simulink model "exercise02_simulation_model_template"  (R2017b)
settings: Solver=ode45  StartTime=0.0  StopTime=10  FixedStep=1e-5  MaxStep=1e-3  RelTol=1e-4  EnableMultiTasking=on
InitFcn:
  | exercise02_simulation_parameters
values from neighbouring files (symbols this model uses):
  cmd_2_newtons_conversion_linear_coefficient = 6.4870e-6    (= 6.487e-06)    [exercise02_get_crazyflie_inner_controller.m]
  cmd_2_newtons_conversion_quadratic_coefficient = 1.3385e-10    [exercise02_get_crazyflie_inner_controller.m]
  cmd_max = 2^16-1    (= 65535)    [exercise02_get_crazyflie_inner_controller.m]
  cmd_min = 0    [exercise02_get_crazyflie_inner_controller.m]
  g = 9.81    [exercise02_get_crazyflie_vehicle_paramters.m]
  K_lqr_outer_loop = K_lqr_outer_loop_discrete_time_200Hz    [exercise02_simulation_parameters.m]
  measurement_noise_accelerometer_covariance_decomposition = U * sqrt(D)    [exercise02_get_measurement_noise_details.m]
  measurement_noise_accelerometer_mean = zeros(3,1)    [exercise02_get_measurement_noise_details.m]
  measurement_noise_accelerometer_seed = randi(measurement_noise_randStream_for_seeds,2^32-1,3,1)    [exercise02_get_measurement_noise_details.m]
  measurement_noise_accelerometer_var = measurement_noise_accelerometer_stddev.^2    [exercise02_get_measurement_noise_details.m]
  measurement_noise_body_accelerations_inclusion_multiplier = 0    [exercise02_get_measurement_noise_details.m]
  measurement_noise_body_rates_inclusion_multiplier = 0    [exercise02_get_measurement_noise_details.m]
  measurement_noise_full_state_covariance_decomposition = U * sqrt(D)    [exercise02_get_measurement_noise_details.m]
  measurement_noise_full_state_inclusion_multiplier = 0    [exercise02_get_measurement_noise_details.m]
  measurement_noise_full_state_mean = [         measurement_noise_p_mean        ;         measurement_noise_p_dot_mean    ;         measurement_noise_psi_mean      ;         measurement_noise_psi_dot_mean        ]    [exercise02_get_measurement_noise_details.m]
  measurement_noise_full_state_seed = [         measurement_noise_p_seed        ;         measurement_noise_p_dot_seed    ;         measurement_noise_psi_seed      ;         measurement_noise_psi_dot_seed        ]    [exercise02_get_measurement_noise_details.m]
  measurement_noise_gyroscope_covariance_decomposition = U * sqrt(D)    [exercise02_get_measurement_noise_details.m]
  measurement_noise_gyroscope_mean = zeros(3,1)    [exercise02_get_measurement_noise_details.m]
  measurement_noise_gyroscope_seed = randi(measurement_noise_randStream_for_seeds,2^32-1,3,1)    [exercise02_get_measurement_noise_details.m]
  measurement_noise_gyroscope_var = measurement_noise_gyroscope_stddev.^2    [exercise02_get_measurement_noise_details.m]
  nrotor_initial_condition = [         nrotor_initial_condition_p          ;         nrotor_initial_condition_p_dot      ;         nrotor_initial_condition_psi        ;         nrotor_initial_condition_psi_dot    ;     ]    [exercise02_get_crazyflie_vehicle_paramters.m]
  nrotor_vehicle_equilibrium_thrust = exercise02_compute_equilibrium_thrusts(nrotor_vehicle_layout_for_controller,nrotor_vehicle_mass_for_controller,g)    [exercise02_simulation_parameters.m]
  nrotor_vehicle_inertia_true = [         16.57 ,   0.83 ,   0.72 ;          0.83 ,  16.66 ,   1.80 ;          0.72 ,   1.80 ,  29.26       ] * 1e-6    [exercise02_get_crazyflie_vehicle_paramters.m]
  nrotor_vehicle_inertia_true_inverse = inv(nrotor_vehicle_inertia_true)    [exercise02_get_crazyflie_vehicle_paramters.m]
  nrotor_vehicle_layout_true = [         [  1 , -1 , -1 ,  1 ] * x_baseline  ;         [ -1 , -1 ,  1 ,  1 ] * y_baseline  ;         [ -1 ,  1 , -1 ,  1 ] * c_baseline        ]    [exercise02_get_crazyflie_vehicle_paramters.m]
  nrotor_vehicle_mass_true = 32e-3    (= 0.032)    [exercise02_get_crazyflie_vehicle_paramters.m]
  nrotor_vehicle_thrust_max = 0.1597*ones( size(nrotor_vehicle_layout_true,2) , 1 )    [exercise02_get_crazyflie_vehicle_paramters.m]
  pid_x_body_rate_integrator_limit = 33.3    [exercise02_get_crazyflie_inner_controller.m]
  pid_x_body_rate_kp = 250.0    (= 250)    [exercise02_get_crazyflie_inner_controller.m]
  pid_y_body_rate_integrator_limit = 33.3    [exercise02_get_crazyflie_inner_controller.m]
  pid_y_body_rate_kp = 250.0    (= 250)    [exercise02_get_crazyflie_inner_controller.m]
  pid_z_body_rate_kp = 120.0    (= 120)    [exercise02_get_crazyflie_inner_controller.m]
  reference_saw_tooth_amplitude_xyz_yaw = [0.3; 0.3; 0.3; 3*deg2rad]    [exercise02_get_reference_specification.m]
  reference_saw_tooth_bias_xyz_yaw = [0.0; 0.0; 0.0; 0*deg2rad]    [exercise02_get_reference_specification.m]
  reference_saw_tooth_inclusion_multiplier = 0    [exercise02_get_reference_specification.m]
  reference_sine_amplitude_xyz_yaw = [0.3; 0.3; 0.3; 3*deg2rad]    [exercise02_get_reference_specification.m]
  reference_sine_bias_xyz_yaw = [0.0; 0.0; 0.0; 0*deg2rad]    [exercise02_get_reference_specification.m]
  reference_sine_period = 5    [exercise02_get_reference_specification.m]
  reference_sine_wave_inclusion_multiplier = 0    [exercise02_get_reference_specification.m]
  reference_step_inclusion_multiplier = 0    [exercise02_get_reference_specification.m]
  reference_step_period = 5    [exercise02_get_reference_specification.m]
  reference_step_xyz_yaw = [0.5; 0.5; 0.5; 10*deg2rad]    [exercise02_get_reference_specification.m]
  sample_time_controller_inner = 1/500    (= 0.002)    [exercise02_simulation_parameters.m]
  sample_time_controller_outer = 1/200    (= 0.005)    [exercise02_simulation_parameters.m]
  sample_time_measurements_body_accelerations = 1/500    (= 0.002)    [exercise02_simulation_parameters.m]
  sample_time_measurements_body_rates = 1/500    (= 0.002)    [exercise02_simulation_parameters.m]
  sample_time_measurements_full_state = 1/200    (= 0.005)    [exercise02_simulation_parameters.m]
undefined symbols (not defined in the file or in its folder): DiscIntNeverNeededParam, sigbuilder_block
libraries: simulink x3
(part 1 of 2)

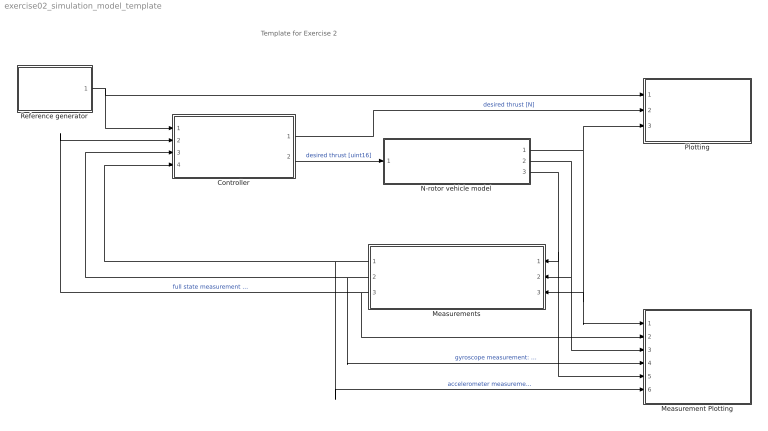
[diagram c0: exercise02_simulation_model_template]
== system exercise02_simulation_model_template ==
  note: Template for Exercise 2
  Controller : Subsystem
  Measurement Plotting : Subsystem
  Measurements : Subsystem
  N-rotor vehicle model : Subsystem
  Plotting : Subsystem
  Reference generator : Subsystem
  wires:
  Controller/1(thrust [N]) -> Plotting/2(thrusts)  "desired thrust [N]"
  N-rotor vehicle model/1(full state) -> Measurement Plotting/1(full state), Measurements/3(full state), Plotting/3(full state)
  Reference generator/1(x,y,z,yaw reference) -> Controller/1(reference), Plotting/1(reference)
  N-rotor vehicle model/2(body rates) -> Measurement Plotting/3(gyroscope), Measurements/2(body rates)
  N-rotor vehicle model/3(accelerations (body frame)) -> Measurement Plotting/5(accelerometer), Measurements/1(acceleration (body frame))
  Measurements/3(full state measurements) -> Controller/2(full state estimate), Measurement Plotting/2(full state measurements)  "full state measurement ( x,y,z , x_dot,y_dot,z_dot , roll,pitch,yaw , roll_dot,pitch_dot,yaw_dot )"
  Measurements/1(accelerometer measurements) -> Controller/4(body accelerations estimate), Measurement Plotting/6(accelerometer measurements)  "accelerometer measurement: ( x,y,z body accelerations )"
  Measurements/2(gyroscope measurements) -> Controller/3(body rates estimate), Measurement Plotting/4(gyroscope measurements)  "gyroscope measurement: ( x,y,z body rates )"
  Controller/2(cmd [uint16]) -> N-rotor vehicle model/1(cmd [uint16])  "desired thrust [uint16]"

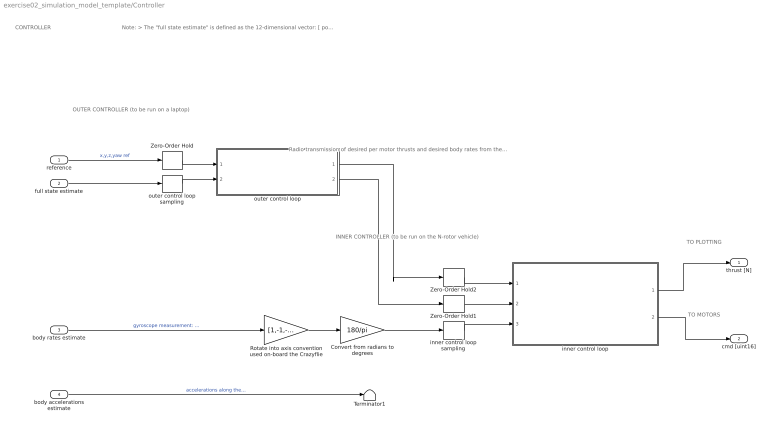
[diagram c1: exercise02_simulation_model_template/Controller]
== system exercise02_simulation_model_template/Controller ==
  note: CONTROLLER
  note: Note: > The "full state estimate" is defined as the 12-dimensional vector: [ position ; velocity ; euler angles ; euler rates ] > The "body rates estimate" is defined as a 3-dimensional vector: angular rate about the body frame [ x ; y ; z ] axes > The "body accelerations estimate" is defined as a 3-dimensional vector: acceleration along the body frame [ x ; y ; z ] axes > The "reference" input is as column vector of length four, specifying in order the reference for each of (x,y,z) position and the yaw euler angle. > The "per motor thrusts [N]" should be output as a column vector with length equal to the number of propellers on the vehicle, i.e., with length equal to N > The "per motor cmd [uint16]" should be output as a column vector with length equal to the number of propellers on the vehicle, i.e., with length equal to N
  note: TO PLOTTING
  note: TO MOTORS
  note: Radio transmission of desired per motor thrusts and desired body rates from the "off-board" laptop to the "on-baord" N-rotor vehicle's micro-processor
  note: OUTER CONTROLLER (to be run on a laptop)
  note: INNER CONTROLLER (to be run on the N-rotor vehicle)
  reference : Inport
  full state estimate : Inport  Port=2
  body rates estimate : Inport  Port=3
  body accelerations estimate : Inport  Port=4
  Convert from radians to degrees : Gain  Gain=180/pi
  Rotate into axis convention used on-board the Crazyflie : Gain  Gain=[1,-1,-1]
  Terminator1 : Terminator
  Zero-Order Hold : ZeroOrderHold  SampleTime=sample_time_controller_outer
  Zero-Order Hold1 : ZeroOrderHold  SampleTime=sample_time_controller_inner
  Zero-Order Hold2 : ZeroOrderHold  SampleTime=sample_time_controller_inner
  inner control loop sampling : ZeroOrderHold  SampleTime=sample_time_controller_inner
  inner control loop : Subsystem
  outer control loop sampling : ZeroOrderHold  SampleTime=sample_time_controller_outer
  outer control loop : Subsystem
  thrust [N] : Outport
  cmd [uint16] : Outport  Port=2
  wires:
  body accelerations estimate/1 -> Terminator1/1  "accelerations along the body frame (x,y,z) axes, in [m / second^2]"
  body rates estimate/1 -> Rotate into axis convention used on-board the Crazyflie/1  "gyroscope measurement: angular rates about the body frame (x,y,z) axes, in [radians / second]"
  inner control loop/1(per motor thrust [N]) -> thrust [N]/1
  reference/1 -> Zero-Order Hold/1  "x,y,z,yaw ref"
  inner control loop/2(per motor cmd [uint16]) -> cmd [uint16]/1
  outer control loop sampling/1 -> outer control loop/2(full state estimate)
  full state estimate/1 -> outer control loop sampling/1
  outer control loop/2(desired body rates [deg/s]) -> Zero-Order Hold1/1
  Rotate into axis convention used on-board the Crazyflie/1 -> Convert from radians to degrees/1
  outer control loop/1(desired per motor thrusts [uint16]) -> Zero-Order Hold2/1
  Convert from radians to degrees/1 -> inner control loop sampling/1
  Zero-Order Hold1/1 -> inner control loop/2(requested body rates [deg/s])
  Zero-Order Hold/1 -> outer control loop/1(reference)
  Zero-Order Hold2/1 -> inner control loop/1(requested per motor comand [uint16])
  inner control loop sampling/1 -> inner control loop/3(body rates estimate [deg/s])

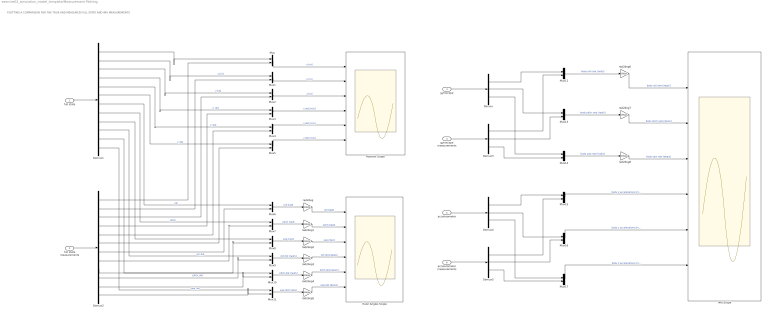
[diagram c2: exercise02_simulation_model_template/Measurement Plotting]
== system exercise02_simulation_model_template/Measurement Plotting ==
  note: PLOTTING A COMPARISON FOR THE TRUE AND MEASURED FULL STATE AND IMU MEASUREMENTS
  full state : Inport
  full state measurements : Inport  Port=2
  gyroscope : Inport  Port=3
  gyroscope measurements : Inport  Port=4
  accelerometer : Inport  Port=5
  accelerometer measurements : Inport  Port=6
  Demux{,3..5} (4 alike) : Demux  Outputs=3
  Demux1 : Demux  Outputs=12
  Demux2 : Demux  Outputs=12
  Euler Angles Scope : Scope  NumInputPorts=6
  IMU Scope : Scope  NumInputPorts=6
  Mux{,1..17} (18 alike) : Mux  Inputs=2
  Postiton Scope : Scope  NumInputPorts=6
  rad2deg{,1..8} (9 alike) : Gain  Gain=180/pi
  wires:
  full state/1 -> Demux1/1
  full state measurements/1 -> Demux2/1
  Mux/1 -> Postiton Scope/1  "x [m]"
  Mux1/1 -> Postiton Scope/2  "y [m]"
  Mux2/1 -> Postiton Scope/3  "z [m]"
  Mux3/1 -> Postiton Scope/4  "x dot [m/s]"
  Mux4/1 -> Postiton Scope/5  "y dot [m/s]"
  Mux5/1 -> Postiton Scope/6  "z dot [m/s]"
  Mux6/1 -> rad2deg/1  "roll [rad]"
  Mux7/1 -> rad2deg1/1  "pitch [rad]"
  Mux8/1 -> rad2deg2/1  "yaw [rad]"
  Mux9/1 -> rad2deg3/1  "roll dot [rad/s]"
  Mux10/1 -> rad2deg4/1  "pitch dot [rad/s]"
  Mux11/1 -> rad2deg5/1  "yaw dot [rad/s]"
  rad2deg/1 -> Euler Angles Scope/1  "roll [deg]"
  rad2deg2/1 -> Euler Angles Scope/3  "yaw [deg]"
  rad2deg1/1 -> Euler Angles Scope/2  "pitch [deg]"
  rad2deg3/1 -> Euler Angles Scope/4  "roll dot [deg/s]"
  rad2deg4/1 -> Euler Angles Scope/5  "pitch dot [deg/s]"
  rad2deg5/1 -> Euler Angles Scope/6  "yaw dot [deg/s]"
  Demux1/1 -> Mux/1
  Demux2/1 -> Mux/2
  Demux1/2 -> Mux1/1  "y [m]"
  Demux1/3 -> Mux2/1  "z [m]"
  Demux2/2 -> Mux1/2
  Demux2/3 -> Mux2/2
  Demux1/4 -> Mux3/1  "x_dot"
  Demux1/5 -> Mux4/1  "y_dot"
  Demux1/6 -> Mux5/1  "z_dot"
  Demux1/12 -> Mux11/1  "yaw_dot"
  Demux1/11 -> Mux10/1  "pitch_dot"
  Demux1/10 -> Mux9/1  "rol_dot"
  Demux1/9 -> Mux8/1
  Demux1/8 -> Mux7/1  "pitch"
  Demux1/7 -> Mux6/1  "roll"
  Demux2/4 -> Mux3/2
  Demux2/5 -> Mux4/2
  Demux2/6 -> Mux5/2
  Demux2/7 -> Mux6/2
  Demux2/8 -> Mux7/2
  Demux2/9 -> Mux8/2
  Demux2/10 -> Mux9/2
  Demux2/11 -> Mux10/2
  Demux2/12 -> Mux11/2
  gyroscope measurements/1 -> Demux3/1
  gyroscope/1 -> Demux/1
  Mux12/1 -> rad2deg6/1  "body roll rate [rad/s]"
  rad2deg6/1 -> IMU Scope/1  "body roll rate [deg/s]"
  Mux13/1 -> rad2deg7/1  "body pitch rate [rad/s]"
  rad2deg7/1 -> IMU Scope/2  "body pitch rate [deg/s]"
  Mux14/1 -> rad2deg8/1  "body yaw rate [rad/s]"
  rad2deg8/1 -> IMU Scope/3  "body yaw rate [deg/s]"
  Demux/1 -> Mux12/1
  Demux/2 -> Mux13/1
  Demux/3 -> Mux14/1
  Demux3/3 -> Mux14/2
  Demux3/2 -> Mux13/2
  Demux3/1 -> Mux12/2
  accelerometer measurements/1 -> Demux5/1
  accelerometer/1 -> Demux4/1
  Mux15/1 -> IMU Scope/4  "body x accelerations [m/s^2]"
  Mux16/1 -> IMU Scope/5  "body y accelerations [m/s^2]"
  Mux17/1 -> IMU Scope/6  "body z accelerations [m/s^2]"
  Demux4/1 -> Mux15/1
  Demux4/2 -> Mux16/1
  Demux4/3 -> Mux17/1
  Demux5/3 -> Mux17/2
  Demux5/2 -> Mux16/2
  Demux5/1 -> Mux15/2

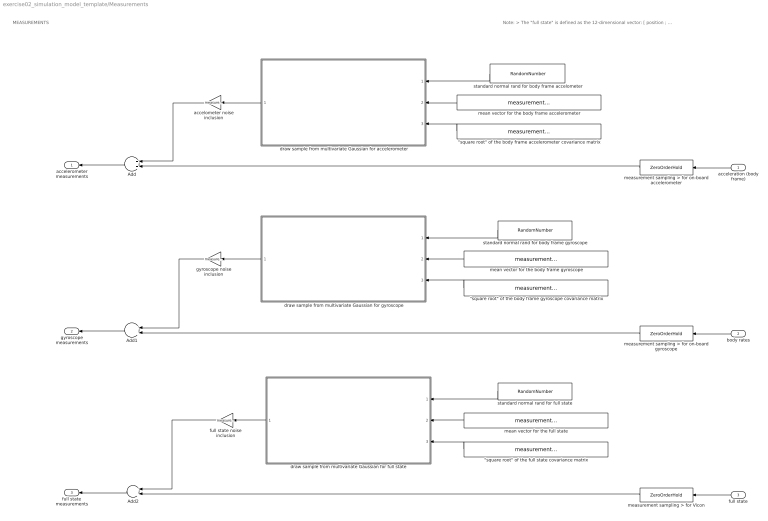
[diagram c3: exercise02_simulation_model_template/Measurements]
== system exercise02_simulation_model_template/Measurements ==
  note: Note: > The "full state" is defined as the 12-dimensional vector: [ position ; velocity ; euler angles ; euler rates ]
  note: MEASUREMENTS
  acceleration (body frame) : Inport
  body rates : Inport  Port=2
  full state : Inport  Port=3
  "\"square root\" of the body frame accelerometer covariance matrix" : Constant  Value=measurement_noise_accelerometer_covariance_decomposition
  "\"square root\" of the body frame gyroscope covariance matrix" : Constant  Value=measurement_noise_gyroscope_covariance_decomposition
  "\"square root\" of the full state covariance matrix" : Constant  Value=measurement_noise_full_state_covariance_decomposition
  Add : Sum
  Add1 : Sum
  Add2 : Sum
  accelometer noise inclusion : Gain  Gain=measurement_noise_body_accelerations_inclusion_multiplier
  draw sample from multivariate Gaussian for accelerometer : MATLAB Function  TreatAsAtomicUnit=on
  draw sample from multivariate Gaussian for full state : MATLAB Function  TreatAsAtomicUnit=on
  draw sample from multivariate Gaussian for gyroscope : MATLAB Function  TreatAsAtomicUnit=on
  full state noise inclusion : Gain  Gain=measurement_noise_full_state_inclusion_multiplier
  gyroscope noise inclusion : Gain  Gain=measurement_noise_body_rates_inclusion_multiplier
  mean vector for the body frame accelerometer : Constant  Value=measurement_noise_accelerometer_mean
  mean vector for the body frame gyroscope : Constant  Value=measurement_noise_gyroscope_mean
  mean vector for the full state : Constant  Value=measurement_noise_full_state_mean
  measurement sampling > for Vicon : ZeroOrderHold  SampleTime=sample_time_measurements_full_state
  measurement sampling > for on-board accelerometer : ZeroOrderHold  SampleTime=sample_time_measurements_body_accelerations
  measurement sampling > for on-board gyroscope : ZeroOrderHold  SampleTime=sample_time_measurements_body_rates
  standard normal rand for body frame accelometer : RandomNumber  Mean=measurement_noise_accelerometer_mean  Variance=measurement_noise_accelerometer_var  Seed=measurement_noise_accelerometer_seed  SampleTime=sample_time_measurements_body_accelerations  VectorParams1D=off
  standard normal rand for body frame gyroscope : RandomNumber  Mean=measurement_noise_gyroscope_mean  Variance=measurement_noise_gyroscope_var  Seed=measurement_noise_gyroscope_seed  SampleTime=sample_time_measurements_body_rates  VectorParams1D=off
  standard normal rand for full state : RandomNumber  Mean=zeros(12,1)  Variance=ones(12,1)  Seed=measurement_noise_full_state_seed  SampleTime=sample_time_measurements_full_state  VectorParams1D=off
  accelerometer measurements : Outport
  gyroscope measurements : Outport  Port=2
  full state measurements : Outport  Port=3
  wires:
  full state/1 -> measurement sampling > for Vicon/1
  acceleration (body frame)/1 -> measurement sampling > for on-board accelerometer/1
  body rates/1 -> measurement sampling > for on-board gyroscope/1
  measurement sampling > for Vicon/1 -> Add2/2
  "\"square root\" of the full state covariance matrix"/1 -> draw sample from multivariate Gaussian for full state/3(covariance_matrix_decomposition)
  mean vector for the full state/1 -> draw sample from multivariate Gaussian for full state/2(mean_vector)
  mean vector for the body frame gyroscope/1 -> draw sample from multivariate Gaussian for gyroscope/2(mean_vector)
  gyroscope noise inclusion/1 -> Add1/1
  measurement sampling > for on-board accelerometer/1 -> Add/2
  mean vector for the body frame accelerometer/1 -> draw sample from multivariate Gaussian for accelerometer/2(mean_vector)
  draw sample from multivariate Gaussian for accelerometer/1(rand_sample) -> accelometer noise inclusion/1
  draw sample from multivariate Gaussian for gyroscope/1(rand_sample) -> gyroscope noise inclusion/1
  standard normal rand for full state/1 -> draw sample from multivariate Gaussian for full state/1(std_normal_rand_sample)
  "\"square root\" of the body frame gyroscope covariance matrix"/1 -> draw sample from multivariate Gaussian for gyroscope/3(covariance_matrix_decomposition)
  accelometer noise inclusion/1 -> Add/1
  draw sample from multivariate Gaussian for full state/1(rand_sample) -> full state noise inclusion/1
  full state noise inclusion/1 -> Add2/1
  measurement sampling > for on-board gyroscope/1 -> Add1/2
  standard normal rand for body frame gyroscope/1 -> draw sample from multivariate Gaussian for gyroscope/1(std_normal_rand_sample)
  standard normal rand for body frame accelometer/1 -> draw sample from multivariate Gaussian for accelerometer/1(std_normal_rand_sample)
  Add2/1 -> full state measurements/1
  "\"square root\" of the body frame accelerometer covariance matrix"/1 -> draw sample from multivariate Gaussian for accelerometer/3(covariance_matrix_decomposition)
  Add/1 -> accelerometer measurements/1
  Add1/1 -> gyroscope measurements/1

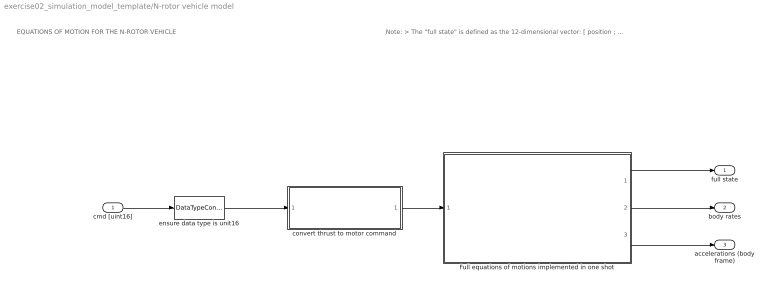
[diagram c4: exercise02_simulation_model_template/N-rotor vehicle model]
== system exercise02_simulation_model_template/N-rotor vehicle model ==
  note: Note: > The "full state" is defined as the 12-dimensional vector: [ position ; velocity ; euler angles ; euler rates ] > The "thrust [N]" input should be a column vector with length equal to the number of propellers on the vehicle, i.e., with length equal to N
  note: EQUATIONS OF MOTION FOR THE N-ROTOR VEHICLE
  cmd [uint16] : Inport
  Full equations of motions implemented in one shot : Subsystem
  convert thrust to motor command : Subsystem
  ensure data type is unit16 : DataTypeConversion  OutDataTypeStr=uint16
  full state : Outport
  body rates : Outport  Port=2
  accelerations (body frame) : Outport  Port=3
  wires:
  cmd [uint16]/1 -> ensure data type is unit16/1
  Full equations of motions implemented in one shot/1(full state) -> full state/1
  Full equations of motions implemented in one shot/2(body rates) -> body rates/1
  Full equations of motions implemented in one shot/3(body accellerations) -> accelerations (body frame)/1
  convert thrust to motor command/1(thrust [N]) -> Full equations of motions implemented in one shot/1(thrusts [N])
  ensure data type is unit16/1 -> convert thrust to motor command/1(cmd [uint16])

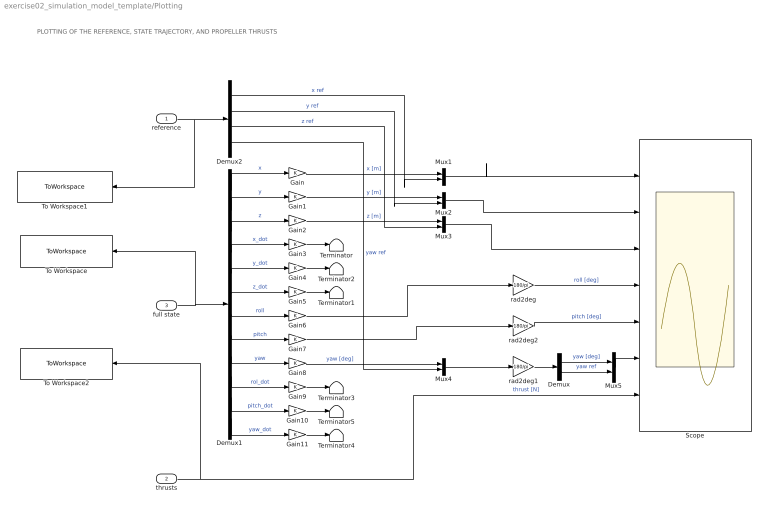
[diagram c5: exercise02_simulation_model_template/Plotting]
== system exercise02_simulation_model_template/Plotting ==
  note: PLOTTING OF THE REFERENCE, STATE TRAJECTORY, AND PROPELLER THRUSTS
  reference : Inport
  thrusts : Inport  Port=2
  full state : Inport  Port=3
  Demux : Demux  Outputs=2
  Demux1 : Demux  Outputs=12
  Demux2 : Demux
  Gain{,1..11} (12 alike) : Gain
  Mux{1..5} (5 alike) : Mux  Inputs=2
  Scope : Scope  NumInputPorts=7
  Terminator{,1..5} (6 alike) : Terminator
  To Workspace : ToWorkspace  VariableName=simout_full_state  SaveFormat=Timeseries  SampleTime=-1
  To Workspace1 : ToWorkspace  VariableName=simout_reference  SaveFormat=Timeseries  SampleTime=-1
  To Workspace2 : ToWorkspace  VariableName=simout_thrusts  SaveFormat=Timeseries  SampleTime=-1
  rad2deg : Gain  Gain=180/pi
  rad2deg1 : Gain  Gain=180/pi
  rad2deg2 : Gain  Gain=180/pi
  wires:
  Demux1/1 -> Gain/1  "x"
  Demux1/2 -> Gain1/1  "y"
  Demux1/6 -> Gain5/1  "z_dot"
  Gain7/1 -> rad2deg2/1
  Demux1/8 -> Gain7/1  "pitch"
  full state/1 -> To Workspace/1, Demux1/1
  Demux1/5 -> Gain4/1  "y_dot"
  Demux1/7 -> Gain6/1  "roll"
  Demux1/4 -> Gain3/1  "x_dot"
  Demux1/3 -> Gain2/1  "z"
  Gain6/1 -> rad2deg/1
  Demux1/9 -> Gain8/1  "yaw"
  Demux1/10 -> Gain9/1  "rol_dot"
  Demux1/11 -> Gain10/1  "pitch_dot"
  Demux1/12 -> Gain11/1  "yaw_dot"
  Gain9/1 -> Terminator3/1
  Gain10/1 -> Terminator5/1
  Gain11/1 -> Terminator4/1
  Gain3/1 -> Terminator/1
  Gain4/1 -> Terminator2/1
  Gain5/1 -> Terminator1/1
  thrusts/1 -> To Workspace2/1, Scope/7  "thrust [N]"
  reference/1 -> To Workspace1/1, Demux2/1
  Mux1/1 -> Scope/1
  Mux2/1 -> Scope/2
  Gain/1 -> Mux1/1  "x [m]"
  Demux2/1 -> Mux1/2  "x ref"
  Gain1/1 -> Mux2/1  "y [m]"
  Demux2/2 -> Mux2/2  "y ref"
  Mux3/1 -> Scope/3
  Gain2/1 -> Mux3/1  "z [m]"
  Demux2/3 -> Mux3/2  "z ref"
  Mux4/1 -> rad2deg1/1
  Gain8/1 -> Mux4/1  "yaw [deg]"
  Demux2/4 -> Mux4/2  "yaw ref"
  rad2deg/1 -> Scope/4  "roll [deg]"
  rad2deg2/1 -> Scope/5  "pitch [deg]"
  Demux/1 -> Mux5/1  "yaw [deg]"
  Demux/2 -> Mux5/2  "yaw ref"
  rad2deg1/1 -> Demux/1
  Mux5/1 -> Scope/6

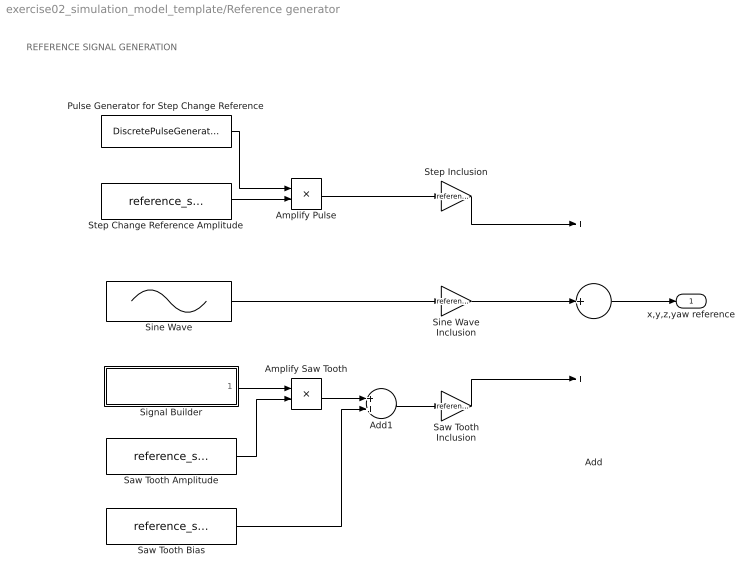
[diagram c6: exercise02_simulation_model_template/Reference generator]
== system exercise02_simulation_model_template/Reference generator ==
  note: REFERENCE SIGNAL GENERATION
  Add : Sum  Inputs=+++
  Add1 : Sum
  Amplify Pulse : Product
  Amplify Saw Tooth : Product
  Pulse Generator for Step Change Reference : DiscretePulseGenerator  PulseType=Time based  Period=reference_step_period*2  PulseWidth=50
  Saw Tooth Amplitude : Constant  Value=reference_saw_tooth_amplitude_xyz_yaw
  Saw Tooth Bias : Constant  Value=reference_saw_tooth_bias_xyz_yaw
  Saw Tooth Inclusion : Gain  Gain=reference_saw_tooth_inclusion_multiplier
  Signal Builder : Subsystem  Tag=STV Subsys  LoadFcn=sigbuilder_block('load');  StartFcn=sigbuilder_block('start');  StopFcn=sigbuilder_block('stop');  ClipboardFcn=sigbuilder_block('clipboard');  mask(Sigbuilder block){tuvar=[0:10]}
      mask help: Simulink:masks:SigbuilderBlock_MD
      mask init:
      | if ~strcmp(get_param(bdroot(gcbh),'SimulationStatus'),'stopped') tuvar = sigbuilder_block('maskInit'); end
  Sine Wave : Sin  Amplitude=reference_sine_amplitude_xyz_yaw  Bias=reference_sine_bias_xyz_yaw  Frequency=2*pi()/reference_sine_period  SampleTime=0
  Sine Wave Inclusion : Gain  Gain=reference_sine_wave_inclusion_multiplier
  Step Change Reference Amplitude : Constant  Value=reference_step_xyz_yaw
  Step Inclusion : Gain  Gain=reference_step_inclusion_multiplier
  x,y,z,yaw reference : Outport
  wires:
  Step Change Reference Amplitude/1 -> Amplify Pulse/2
  Pulse Generator for Step Change Reference/1 -> Amplify Pulse/1
  Sine Wave/1 -> Sine Wave Inclusion/1
  Add/1 -> x,y,z,yaw reference/1
  Step Inclusion/1 -> Add/1
  Sine Wave Inclusion/1 -> Add/2
  Amplify Pulse/1 -> Step Inclusion/1
  Saw Tooth Inclusion/1 -> Add/3
  Signal Builder/1(Saw Tooth) -> Amplify Saw Tooth/1
  Saw Tooth Amplitude/1 -> Amplify Saw Tooth/2
  Amplify Saw Tooth/1 -> Add1/1
  Add1/1 -> Saw Tooth Inclusion/1
  Saw Tooth Bias/1 -> Add1/2

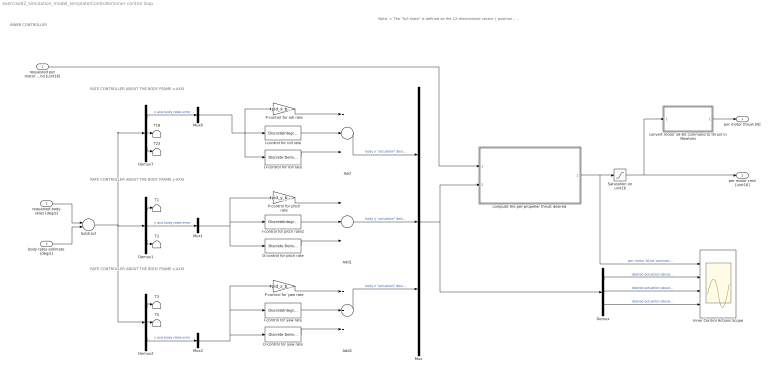
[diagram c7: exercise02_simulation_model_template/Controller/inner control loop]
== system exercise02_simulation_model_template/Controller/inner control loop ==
  note: RATE CONTROLLER ABOUT THE BODY FRAME z-AXIS
  note: RATE CONTROLLER ABOUT THE BODY FRAME y-AXIS
  note: RATE CONTROLLER ABOUT THE BODY FRAME x-AXIS
  note: INNER CONTROLLER
  note: Note: > The "full state" is defined as the 12-dimensional vector: [ position ; velocity ; euler angles ; euler rates ] > The "thrusts ref" is input as a column vector with a desired 16-bit command per motor, i.e., with length equal to N
  requested per motor comand [uint16] : Inport
  requested body rates [deg/s] : Inport  Port=2
  body rates estimate [deg/s] : Inport  Port=3
  Add : Sum  Inputs=+++
  Add1 : Sum  Inputs=+++
  Add2 : Sum  Inputs=+++
  D-control for pitch rate : simulink/Discrete/Discrete Derivative  gainval=pid_y_body_rate_kd  ICPrevScaledInput=0.0  OutMin=[]  OutMax=[]  OutDataType=fixdt(1, 16)  OutScaling=2^-10  DoSatur=off
  D-control for roll rate : simulink/Discrete/Discrete Derivative  gainval=pid_x_body_rate_kd  ICPrevScaledInput=0.0  OutMin=[]  OutMax=[]  OutDataType=fixdt(1, 16)  OutScaling=2^-10  DoSatur=off
  D-control for yaw rate : simulink/Discrete/Discrete Derivative  gainval=pid_z_body_rate_kd  ICPrevScaledInput=0.0  OutMin=[]  OutMax=[]  OutDataType=fixdt(1, 16)  OutScaling=2^-10  DoSatur=off
  Demux{,1..2,7} (4 alike) : Demux  Outputs=3
  I-control for pitch rate2 : DiscreteIntegrator  gainval=pid_y_body_rate_ki  InitialConditionSetting=State (most efficient)  SampleTime=-1  LimitOutput=on  UpperSaturationLimit=pid_y_body_rate_integrator_limit  LowerSaturationLimit=-pid_y_body_rate_integrator_limit  ICPrevOutput=DiscIntNeverNeededParam  ICPrevScaledInput=DiscIntNeverNeededParam
  I-control for roll rate : DiscreteIntegrator  gainval=pid_x_body_rate_ki  InitialConditionSetting=State (most efficient)  SampleTime=-1  LimitOutput=on  UpperSaturationLimit=pid_x_body_rate_integrator_limit  LowerSaturationLimit=-pid_x_body_rate_integrator_limit  ICPrevOutput=DiscIntNeverNeededParam  ICPrevScaledInput=DiscIntNeverNeededParam
  I-control for yaw rate : DiscreteIntegrator  gainval=pid_z_body_rate_ki  InitialConditionSetting=State (most efficient)  SampleTime=-1  LimitOutput=on  UpperSaturationLimit=pid_x_body_rate_integrator_limit  LowerSaturationLimit=-pid_x_body_rate_integrator_limit  ICPrevOutput=DiscIntNeverNeededParam  ICPrevScaledInput=DiscIntNeverNeededParam
  Inner Control Actions Scope : Scope  NumInputPorts=4
  Mux : Mux  Inputs=3
  Mux1 : Mux  Inputs=1
  Mux2 : Mux  Inputs=1
  Mux6 : Mux  Inputs=1
  P-control for pitch rate : Gain  Gain=pid_y_body_rate_kp
  P-control for roll rate : Gain  Gain=pid_x_body_rate_kp
  P-control for yaw rate : Gain  Gain=pid_z_body_rate_kp
  Saturation on uint16 : Saturate  UpperLimit=cmd_max  LowerLimit=cmd_min  ZeroCross=off
  Subtract : Sum  Inputs=+-
  T{1..3,5,18,23} (6 alike) : Terminator
  compute the per-propeller thrust desired : MATLAB Function  TreatAsAtomicUnit=on
  convert motor 16-bit command to thrust in Newtons : Subsystem
  per motor thrust [N] : Outport
  per motor cmd [uint16] : Outport  Port=2
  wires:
  compute the per-propeller thrust desired/1(cmd_to_apply) -> Inner Control Actions Scope/1, Saturation on uint16/1  "per motor 16-bit command after distribute power function [uint16]"
  body rates estimate [deg/s]/1 -> Subtract/2
  requested per motor comand [uint16]/1 -> compute the per-propeller thrust desired/1(cmd_per_motor_desired)
  requested body rates [deg/s]/1 -> Subtract/1
  Add/1 -> Mux/1  "body x \"actuation\" desired [uint16]"
  Add1/1 -> Mux/2  "body y \"actuation\" desired [uint16]"
  Add2/1 -> Mux/3  "body z \"actuation\" desired [uint16]"
  Subtract/1 -> Demux2/1, Demux1/1, Demux7/1
  Mux/1 -> Demux/1, compute the per-propeller thrust desired/2(cmd_for_body_torques_desired)
  Saturation on uint16/1 -> per motor cmd [uint16]/1, convert motor 16-bit command to thrust in Newtons/1(cmd [uint16])
  Demux/1 -> Inner Control Actions Scope/2  "desired actuation about body frame x axis [uint16]"
  Demux/2 -> Inner Control Actions Scope/3  "desired actuation about body frame x axis [uint16]"
  Demux/3 -> Inner Control Actions Scope/4  "desired actuation about body frame x axis [uint16]"
  Demux7/2 -> T18/1
  Mux6/1 -> P-control for roll rate/1, I-control for roll rate/1, D-control for roll rate/1
  Demux7/3 -> T23/1
  Demux7/1 -> Mux6/1  "x axis body rates error"
  Demux1/2 -> Mux1/1  "y axis body rates error"
  Demux1/3 -> T2/1
  Demux1/1 -> T1/1
  Demux2/3 -> Mux2/1  "z axis body rates error"
  Demux2/1 -> T3/1
  Mux2/1 -> I-control for yaw rate/1, P-control for yaw rate/1, D-control for yaw rate/1
  Demux2/2 -> T5/1
  convert motor 16-bit command to thrust in Newtons/1(thrusts [N]) -> per motor thrust [N]/1
  P-control for roll rate/1 -> Add/1
  I-control for roll rate/1 -> Add/2
  D-control for roll rate/1 -> Add/3
  P-control for pitch rate/1 -> Add1/1
  I-control for pitch rate2/1 -> Add1/2
  D-control for pitch rate/1 -> Add1/3
  Mux1/1 -> D-control for pitch rate/1, P-control for pitch rate/1, I-control for pitch rate2/1
  D-control for yaw rate/1 -> Add2/3
  P-control for yaw rate/1 -> Add2/1
  I-control for yaw rate/1 -> Add2/2

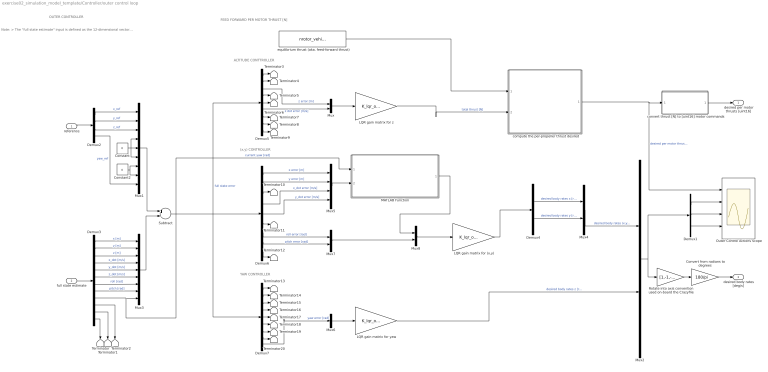
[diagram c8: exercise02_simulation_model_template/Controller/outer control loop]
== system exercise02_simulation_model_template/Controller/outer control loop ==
  note: FEED FORWARD PER MOTOR THRUST [N]
  note: YAW CONTROLLER
  note: (x,y) CONTROLLER
  note: ALTITUDE CONTTROLLER
  note: OUTER CONTROLLER
  note: Note: > The "full state estimate" input is defined as the 12-dimensional vector: [ position ; velocity ; euler angles ; euler rates ] > The "reference" input is as column vector of length four, specifying in order the reference for each of (x,y,z) position and the yaw euler angle. > The "desired per motor thrusts" output as a column vector with length equal to the number of propellers, i.e., with length equal to N. > The "desired body rates" output should be a column vector of length 3 (i.e., the desired angular rates about the body frame x,y, and z axes).
  reference : Inport
  full state estimate : Inport  Port=2
  Constant : Constant  Value=0
  Constant2 : Constant  Value=0
  Convert from radians to degrees : Gain  Gain=180/pi
  Demux1 : Demux  Outputs=3
  Demux2 : Demux
  Demux3 : Demux  Outputs=12
  Demux4 : Demux  Outputs=2
  Demux5 : Demux  Outputs=9
  Demux6 : Demux  Outputs=9
  Demux7 : Demux  Outputs=9
  LQR gain matrix for (x,y) : Gain  Gain=K_lqr_outer_loop(2:3,[1,2,4,5,7,8])  Multiplication=Matrix(K*u)
  LQR gain matrix for yaw : Gain  Gain=K_lqr_outer_loop(4,9)  Multiplication=Matrix(K*u)
  LQR gain matrix for z : Gain  Gain=K_lqr_outer_loop(1,[3,6])  Multiplication=Matrix(K*u)
  MATLAB Function : MATLAB Function  TreatAsAtomicUnit=on
  Mux{,2,4,7..8} (5 alike) : Mux  Inputs=2
  Mux1 : Mux  Inputs=9
  Mux3 : Mux  Inputs=9
  Mux5 : Mux
  Mux6 : Mux  Inputs=1
  Outer Control Actions Scope : Scope  NumInputPorts=4
  Rotate into axis convention used on-board the Crazyflie : Gain  Gain=[1,-1,-1]
  Subtract : Sum  Inputs=+-
  Terminator{,1..20} (21 alike) : Terminator
  compute the per-propeller thrust desired : MATLAB Function  TreatAsAtomicUnit=on
  convert thrust [N] to [uint16] motor commands : Subsystem
  equilibrium thrust (aka. feed-forward thrust) : Constant  Value=nrotor_vehicle_equilibrium_thrust
  desired per motor thrusts [uint16] : Outport
  desired body rates [deg/s] : Outport  Port=2
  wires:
  Mux1/1 -> Subtract/1
  reference/1 -> Demux2/1
  Demux2/1 -> Mux1/1  "x_ref"
  equilibrium thrust (aka. feed-forward thrust)/1 -> compute the per-propeller thrust desired/1(thrusts_for_equilibrium)
  Constant2/1 -> Mux1/8, Mux1/7
  Demux2/3 -> Mux1/3  "z_ref"
  Demux2/2 -> Mux1/2  "y_ref"
  Demux2/4 -> Mux1/9  "yaw_ref"
  Constant/1 -> Mux1/6, Mux1/4, Mux1/5
  LQR gain matrix for z/1 -> compute the per-propeller thrust desired/2(additional_thrust_desired)  "total thrust [N]"
  compute the per-propeller thrust desired/1(thrusts_per_motor) -> convert thrust [N] to [uint16] motor commands/1(thrust [N]), Outer Control Actions Scope/1  "desired per motor thrusts [N]"
  full state estimate/1 -> Demux3/1
  Demux3/1 -> Mux3/1  "x [m]"
  Demux3/2 -> Mux3/2  "y [m]"
  Demux3/3 -> Mux3/3  "z [m]"
  Demux3/4 -> Mux3/4  "x_dot [m/s]"
  Demux3/5 -> Mux3/5  "y_dot [m/s]"
  Demux3/7 -> Mux3/7  "roll [rad]"
  Demux3/6 -> Mux3/6  "z_dot [m/s]"
  Demux3/8 -> Mux3/8  "pitch [rad]"
  Demux3/9 -> MATLAB Function/1(current_yaw), Mux3/9  "current yaw [rad]"
  Demux3/10 -> Terminator2/1
  Demux3/11 -> Terminator1/1
  Demux3/12 -> Terminator/1
  Mux3/1 -> Subtract/2
  Demux1/3 -> Outer Control Actions Scope/4
  Demux1/2 -> Outer Control Actions Scope/3
  Demux1/1 -> Outer Control Actions Scope/2
  Subtract/1 -> Demux7/1, Demux5/1, Demux6/1  "full state error"
  LQR gain matrix for yaw/1 -> Mux2/2  "desired body rates z [rad/s]"
  LQR gain matrix for (x,y)/1 -> Demux4/1
  Demux4/2 -> Mux4/2  "desired body rates y [rad/s]"
  Demux4/1 -> Mux4/1  "desired body rates x [rad/s]"
  Mux4/1 -> Mux2/1  "desired body rates (x,y) [rad/s]"
  Demux5/3 -> Mux/1  "z error [m]"
  Demux5/6 -> Mux/2  "z dot error [m/s]"
  Demux5/1 -> Terminator3/1
  Demux5/2 -> Terminator4/1
  Demux5/4 -> Terminator5/1
  Demux5/5 -> Terminator6/1
  Demux5/7 -> Terminator7/1
  Demux5/8 -> Terminator8/1
  Demux5/9 -> Terminator9/1
  Mux/1 -> LQR gain matrix for z/1
  Demux6/1 -> Mux5/1  "x error [m]"
  Demux6/2 -> Mux5/2  "y error [m]"
  Demux6/4 -> Mux5/3  "x_dot error [m/s]"
  Demux6/5 -> Mux5/4  "y_dot error [m/s]"
  Demux6/7 -> Mux7/1  "roll error [rad]"
  Demux6/8 -> Mux7/2  "pitch error [rad]"
  Demux6/9 -> Terminator12/1
  Mux8/1 -> LQR gain matrix for (x,y)/1
  Demux6/6 -> Terminator11/1
  Demux6/3 -> Terminator10/1
  Demux7/1 -> Terminator13/1
  Demux7/2 -> Terminator14/1
  Demux7/4 -> Terminator16/1
  Demux7/5 -> Terminator17/1
  Demux7/7 -> Terminator19/1
  Demux7/8 -> Terminator20/1
  Demux7/9 -> Mux6/1  "yaw error [rad]"
  Mux6/1 -> LQR gain matrix for yaw/1
  Demux7/3 -> Terminator15/1
  Demux7/6 -> Terminator18/1
  Mux7/1 -> Mux8/2
  Mux5/1 -> MATLAB Function/2(xy_error_in_inertial_frame)
  MATLAB Function/1(xy_error_in_body_frame) -> Mux8/1
  convert thrust [N] to [uint16] motor commands/1(cmd [uint16]) -> desired per motor thrusts [uint16]/1
  Mux2/1 -> Rotate into axis convention used on-board the Crazyflie/1, Demux1/1
  Convert from radians to degrees/1 -> desired body rates [deg/s]/1
  Rotate into axis convention used on-board the Crazyflie/1 -> Convert from radians to degrees/1

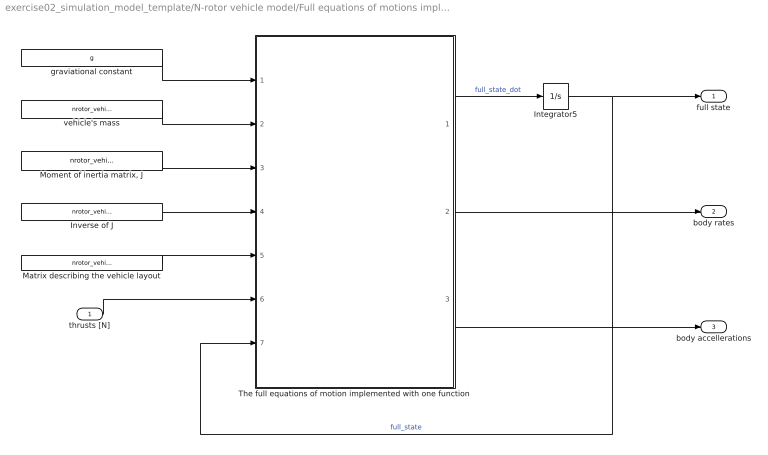
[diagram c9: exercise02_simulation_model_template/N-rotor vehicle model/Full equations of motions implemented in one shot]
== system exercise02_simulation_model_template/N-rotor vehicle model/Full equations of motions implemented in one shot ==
  thrusts [N] : Inport
  Integrator5 : Integrator  InitialCondition=nrotor_initial_condition
  Inverse of J : Constant  Value=nrotor_vehicle_inertia_true_inverse
  Matrix describing the vehicle layout : Constant  Value=nrotor_vehicle_layout_true
  "Moment of inertia matrix, J" : Constant  Value=nrotor_vehicle_inertia_true
  The full equations of motion implemented with one function : MATLAB Function  TreatAsAtomicUnit=on
  graviational constant : Constant  Value=g
  vehicle's mass : Constant  Value=nrotor_vehicle_mass_true
  full state : Outport
  body rates : Outport  Port=2
  body accellerations : Outport  Port=3
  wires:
  The full equations of motion implemented with one function/1(full_state_dot) -> Integrator5/1  "full_state_dot"
  Matrix describing the vehicle layout/1 -> The full equations of motion implemented with one function/5(layout)
  The full equations of motion implemented with one function/3(body_accel) -> body accellerations/1
  graviational constant/1 -> The full equations of motion implemented with one function/1(g)
  thrusts [N]/1 -> The full equations of motion implemented with one function/6(thrusts)
  The full equations of motion implemented with one function/2(body_rates) -> body rates/1
  Integrator5/1 -> full state/1, The full equations of motion implemented with one function/7(full_state)  "full_state"
  Inverse of J/1 -> The full equations of motion implemented with one function/4(J_inv)
  vehicle's mass/1 -> The full equations of motion implemented with one function/2(m)
  "Moment of inertia matrix, J"/1 -> The full equations of motion implemented with one function/3(J)

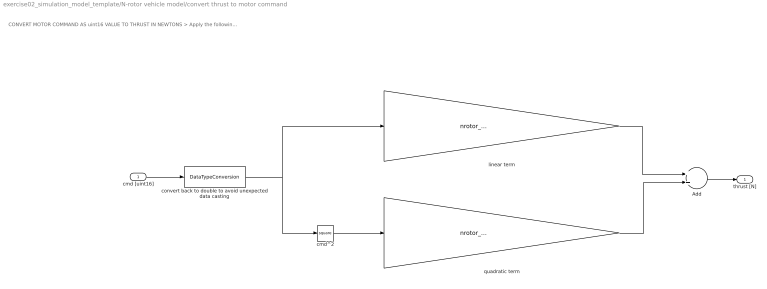
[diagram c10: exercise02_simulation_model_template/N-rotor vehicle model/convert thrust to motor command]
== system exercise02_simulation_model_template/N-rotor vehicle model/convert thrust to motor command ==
  note: CONVERT MOTOR COMMAND AS uint16 VALUE TO THRUST IN NEWTONS > Apply the following equation: thust [N] = nrotor_vehicle_thrust_max * ( cmd_2_newtons_conversion_quadratic_coefficient * cmd^2 + cmd_2_newtons_conversion_linear_coefficient * cmd ) > This sub-system acts element-wise on the input, i.e., the output is a vector of the same length as the input
  cmd [uint16] : Inport
  Add : Sum
  cmd^2 : Math  Operator=square
  convert back to double to avoid unexpected data casting : DataTypeConversion  OutDataTypeStr=double
  linear term : Gain  Gain=nrotor_vehicle_thrust_max .* cmd_2_newtons_conversion_linear_coefficient
  quadratic term : Gain  Gain=nrotor_vehicle_thrust_max .* cmd_2_newtons_conversion_quadratic_coefficient
  thrust [N] : Outport
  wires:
  cmd^2/1 -> quadratic term/1
  quadratic term/1 -> Add/2
  linear term/1 -> Add/1
  cmd [uint16]/1 -> convert back to double to avoid unexpected data casting/1
  Add/1 -> thrust [N]/1
  convert back to double to avoid unexpected data casting/1 -> linear term/1, cmd^2/1

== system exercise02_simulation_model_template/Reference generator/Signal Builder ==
  Demux : Demux  Tag=STV Demux  Outputs=1
  FromWs : FromWorkspace  Tag=STV FromWs  VariableName=tuvar  SampleTime=0
  Saw Tooth : Outport  Tag=STV Outport
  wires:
  Demux/1 -> Saw Tooth/1
  FromWs/1 -> Demux/1

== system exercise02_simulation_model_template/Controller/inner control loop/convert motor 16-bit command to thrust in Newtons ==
  note: CONVERT MOTOR COMMAND AS uint16 VALUE TO THRUST IN NEWTONS > Apply the following equation: thust [N] = nrotor_vehicle_thrust_max * ( cmd_2_newtons_conversion_quadratic_coefficient * cmd^2 + cmd_2_newtons_conversion_linear_coefficient * cmd ) > This sub-system acts element-wise on the input, i.e., the output is a vector of the same length as the input
  cmd [uint16] : Inport
  Add : Sum
  cmd^2 : Math  Operator=square
  convert back to double to avoid unexpected data casting : DataTypeConversion  OutDataTypeStr=double
  linear term : Gain  Gain=nrotor_vehicle_thrust_max .* cmd_2_newtons_conversion_linear_coefficient
  quadratic term : Gain  Gain=nrotor_vehicle_thrust_max .* cmd_2_newtons_conversion_quadratic_coefficient
  thrusts [N] : Outport
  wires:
  cmd^2/1 -> quadratic term/1
  quadratic term/1 -> Add/2
  linear term/1 -> Add/1
  cmd [uint16]/1 -> convert back to double to avoid unexpected data casting/1
  Add/1 -> thrusts [N]/1
  convert back to double to avoid unexpected data casting/1 -> linear term/1, cmd^2/1

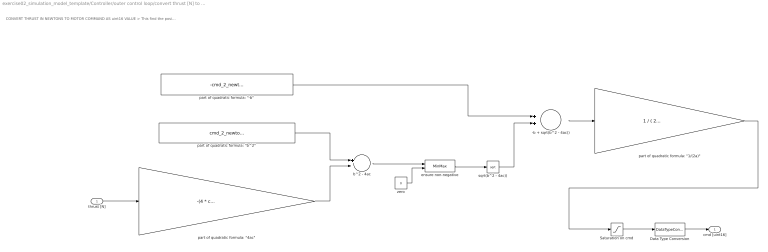
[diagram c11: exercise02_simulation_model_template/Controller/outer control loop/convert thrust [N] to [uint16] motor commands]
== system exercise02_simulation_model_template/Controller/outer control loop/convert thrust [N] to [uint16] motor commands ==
  note: CONVERT THRUST IN NEWTONS TO MOTOR COMMAND AS uint16 VALUE > This find the positive solution of the equation: thust [N] = nrotor_vehicle_thrust_max * ( cmd_2_newtons_conversion_quadratic_coefficient * cmd^2 + cmd_2_newtons_conversion_linear_coefficient * cmd ) > This sub-system acts element-wise on the input, i.e., the output is a vector of the same length as the input
  thrust [N] : Inport
  -b + sqrt(b^2 - 4ac)) : Sum
  Data Type Conversion : DataTypeConversion  OutDataTypeStr=uint16
  Saturation on cmd : Saturate  UpperLimit=cmd_max  LowerLimit=cmd_min  ZeroCross=off
  b^2 - 4ac : Sum  Inputs=+-
  ensure non-negative : MinMax  Function=max  Inputs=2
  "part of quadratic formula: \"-b\"" : Constant  Value=-cmd_2_newtons_conversion_linear_coefficient
  "part of quadratic formula: \"1/(2a)\"" : Gain  Gain=1 / ( 2 * cmd_2_newtons_conversion_quadratic_coefficient )
  "part of quadratic formula: \"4ac\"" : Gain  Gain=-(4 * cmd_2_newtons_conversion_quadratic_coefficient) ./ nrotor_vehicle_thrust_max
  "part of quadratic formula: \"b^2\"" : Constant  Value=cmd_2_newtons_conversion_linear_coefficient^2
  sqrt(b^2 - 4ac)) : Sqrt
  zero : Constant  Value=0
  cmd [uint16] : Outport
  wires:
  thrust [N]/1 -> "part of quadratic formula: \"4ac\""/1
  Saturation on cmd/1 -> Data Type Conversion/1
  Data Type Conversion/1 -> cmd [uint16]/1
  "part of quadratic formula: \"4ac\""/1 -> b^2 - 4ac/2
  "part of quadratic formula: \"b^2\""/1 -> b^2 - 4ac/1
  b^2 - 4ac/1 -> ensure non-negative/1
  ensure non-negative/1 -> sqrt(b^2 - 4ac))/1
  "part of quadratic formula: \"-b\""/1 -> -b + sqrt(b^2 - 4ac))/1
  sqrt(b^2 - 4ac))/1 -> -b + sqrt(b^2 - 4ac))/2
  -b + sqrt(b^2 - 4ac))/1 -> "part of quadratic formula: \"1/(2a)\""/1
  "part of quadratic formula: \"1/(2a)\""/1 -> Saturation on cmd/1
  zero/1 -> ensure non-negative/2

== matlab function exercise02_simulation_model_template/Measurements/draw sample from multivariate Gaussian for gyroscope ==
function rand_sample = mvn_gyroscope( std_normal_rand_sample , mean_vector , covariance_matrix_decomposition )


% Compute the multi-variate Gaussian sample from a distirbution with:
% > "mean_vector" as the mean, and
% > "covariance_matrix_decomposition" as the "square root" of the
%    covariance matrix
rand_sample = mean_vector + covariance_matrix_decomposition * std_normal_rand_sample;

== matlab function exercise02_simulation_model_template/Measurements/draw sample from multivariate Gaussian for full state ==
function rand_sample = mvn_full_state( std_normal_rand_sample , mean_vector , covariance_matrix_decomposition )


% Compute the multi-variate Gaussian sample from a distirbution with:
% > "mean_vector" as the mean, and
% > "covariance_matrix_decomposition" as the "square root" of the
%    covariance matrix
rand_sample = mean_vector + covariance_matrix_decomposition * std_normal_rand_sample;

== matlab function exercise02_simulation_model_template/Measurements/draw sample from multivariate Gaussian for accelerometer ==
function rand_sample = mvn_accelerometer( std_normal_rand_sample , mean_vector , covariance_matrix_decomposition )


% Compute the multi-variate Gaussian sample from a distirbution with:
% > "mean_vector" as the mean, and
% > "covariance_matrix_decomposition" as the "square root" of the
%    covariance matrix
rand_sample = mean_vector + covariance_matrix_decomposition * std_normal_rand_sample;

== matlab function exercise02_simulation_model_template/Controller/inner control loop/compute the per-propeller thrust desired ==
function cmd_to_apply = distribute_power( cmd_per_motor_desired , cmd_for_body_torques_desired )
% ----------------------------------------------------------------------- %
% DESCRIPTION:
% This function computes the uint16 command to apply to each motor as per
% the code that runs "on-board" on the Crazyflie's firmware
%
%
% INPUT ARGUMENTS:
%
% cmd_per_motor_desired [uint16]
% > This is a colulmn vector with length equal to the number of propellers
%   on the Crazyflie, i.e., 4, and each element represents the "baseline"
%   16-bit command that should be requested from the Crazyflie, as
%   requested by the outer loop controller.
%
% cmd_for_body_torques_desired [uint16]
% > This is the "actuation" uint16 command that comes directly from the
%   output of the Crazyflie's body rate PID controllers running in the
%   firmware. This value of command has already been adjust for the
%   dimensions of the Crazyflie, and the pattern for distributing the
%   command across the motor is provided in the exercise sheet.
%
%
% RETURN ARGUMENTS:
% % cmd_to_apply [uint16]
% > This is a colulmn vector with length equal to the number of propellers
%   on the Crazyflie, i.e., 4, and each element represents the 16-bit
%   command that will be requested from the motors
%
%
% DATA FORMAT ASSUMPTIONS:
% > the "cmd_per_motor_desired" vector is such when applied, the static
%   thrusts exert no torque about the body frame axes
%
% ----------------------------------------------------------------------- %


% Get the uint16 commands into a separate variable for each motor
cmd1 = cmd_per_motor_desired(1);
cmd2 = cmd_per_motor_desired(2);
cmd3 = cmd_per_motor_desired(3);
cmd4 = cmd_per_motor_desired(4);


% Get the desired body torques uint16 commands into a separate variable for
% the "uint16 command torque" desired about each of the body frame axes
r = cmd_for_body_torques_desired(1) / 2;
p = cmd_for_body_torques_desired(2) / 2;
y = cmd_for_body_torques_desired(3);


% These variable names have been used to partially match the code from the
% Crazyflie firmware:
% r  -  where "r" stands for roll, this is the "uint16 command torque" to
%       apply about the body-frame's x-axis, i.e., the roll-axis
% p  -  where "p" stands for pitch, this is the "uint16 command torque" to
%       apply about the body-frame's y-axis, i.e., the pitch-axis
% y  -  where "y" stands for yaw, this is the "uint16 command torque" to
%       apply about the body-frame's z-axis, i.e., the yaw-axis
%
% Note: the "/ 2" for the extraction of "r" and "p" above is simply added
% to minimic the code of the Crazyflie firmware. Presumably the Crazyflie's
% PID contollers for the body-frame roll and pitch axis are tuned with this
% factor of "/ 2" appropriately accounted for.


% Initialise the return variable "cmd_to_apply" to zeros
% > This can be required so that Simulink knows the expected size
cmd_to_apply = zeros(4,1);

% Compute the 16-bit command that should be applied from each motor as per
% the code from the Crazyflie firmware
% > For motor 1:
cmd_to_apply(1,1)  =  cmd1   - r   + p  +  y;
% > For motor 1:
cmd_to_apply(2,1)  =  cmd2   - r   - p  -  y;
% > For motor 1:
cmd_to_apply(3,1)  =  cmd3   + r   - p  +  y;
% > For motor 1:
cmd_to_apply(4,1)  =  cmd4   + r   + p  -  y;
